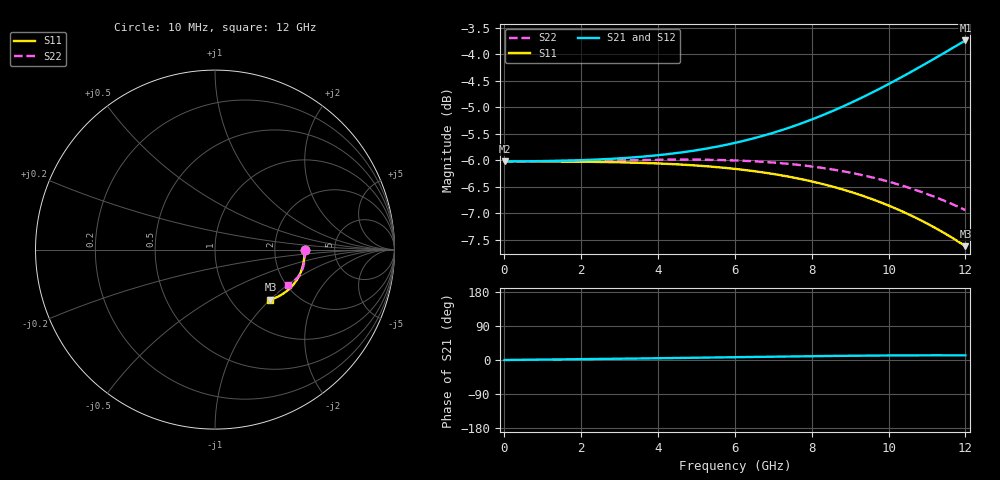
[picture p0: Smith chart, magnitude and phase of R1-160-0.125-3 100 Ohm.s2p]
!version-2
!date-03.2021
# MHz S RI R 50
!Freq ReS11 ImS11 ReS21 ImS21 ReS12 ImS12 ReS22 ImS22
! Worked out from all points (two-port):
!   601 points, 10 MHz to 12 GHz, reference 50 ohm
!   highest |S21| = -3.74 dB at 12 GHz (marker M1); lowest = -6.0 dB at 10 MHz (marker M2)
!   |S21| within 3 dB of the highest: start of sweep to end of sweep
!   lowest |S11| = -7.6 dB at 12 GHz (marker M3), VSWR 2.42, Z = 74.5 - j50.2 ohm
!   |S11| at or under -10 dB: nowhere
!   |S22| runs from -6.9 to -6.0 dB; largest |S21 - S12| = 0
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10  0.5 -0.000214  0.5 9.15e-05  0.5 9.15e-05  0.5 -0.000133
1030  0.4994 -0.0221  0.5002 0.0095  0.5002 0.0095  0.5 -0.0138
2010  0.4977 -0.0435  0.501 0.0189  0.501 0.0189  0.4999 -0.0274
3050  0.4944 -0.0671  0.5026 0.0297  0.5026 0.0297  0.4995 -0.0425
4010  0.4896 -0.0898  0.5051 0.0407  0.5051 0.0407  0.4985 -0.0575
4550  0.4859 -0.103  0.5072 0.0473  0.5072 0.0473  0.4975 -0.0664
5050  0.4817 -0.1156  0.5097 0.0538  0.5097 0.0538  0.4962 -0.0749
5530  0.477 -0.1279  0.5127 0.0602  0.5127 0.0602  0.4946 -0.0834
6010  0.4714 -0.1404  0.5162 0.0669  0.5162 0.0669  0.4924 -0.0921
6530  0.4644 -0.1541  0.5208 0.0743  0.5208 0.0743  0.4895 -0.1018
7030  0.4566 -0.1674  0.5261 0.0816  0.5261 0.0816  0.486 -0.1114
7530  0.4476 -0.1808  0.5323 0.089  0.5323 0.089  0.4818 -0.121
8010  0.4378 -0.1935  0.5392 0.096  0.5392 0.096  0.477 -0.1303
8510  0.4263 -0.2065  0.5474 0.1032  0.5474 0.1032  0.4712 -0.14
9010  0.4135 -0.2192  0.5567 0.1102  0.5567 0.1102  0.4644 -0.1495
9510  0.3994 -0.2314  0.5671 0.1168  0.5671 0.1168  0.4567 -0.1587
10010  0.3838 -0.2429  0.5786 0.1228  0.5786 0.1228  0.4481 -0.1675
10530  0.3662 -0.2539  0.5918 0.1284  0.5918 0.1284  0.4381 -0.1762
11070  0.3464 -0.2642  0.6067 0.1332  0.6067 0.1332  0.4268 -0.1843
11570  0.3268 -0.2724  0.6215 0.1365  0.6215 0.1365  0.4153 -0.1911
11930  0.312 -0.2775  0.6327 0.1383  0.6327 0.1383  0.4066 -0.1953
12000  0.3091 -0.2784  0.635 0.1385  0.635 0.1385  0.4049 -0.1961
